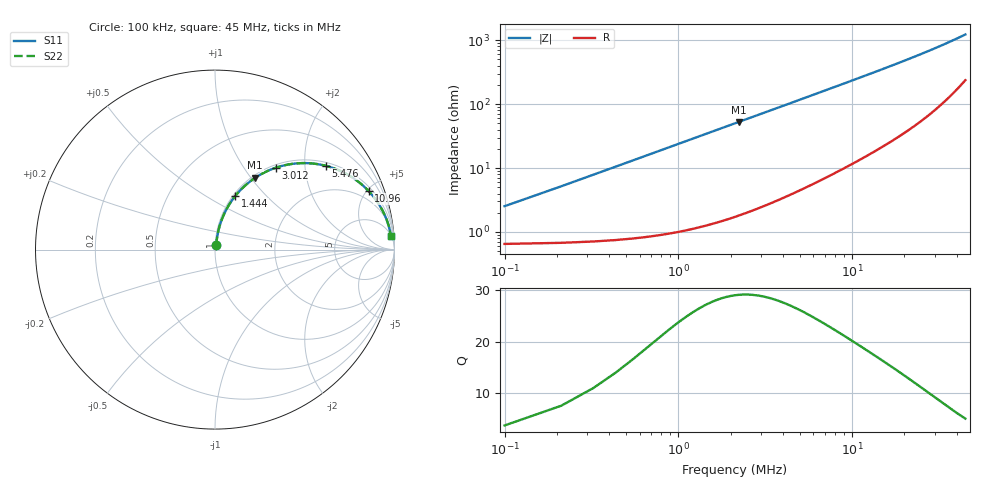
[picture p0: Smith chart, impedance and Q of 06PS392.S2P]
! Coilcraft 0603PS-392 Power Chip Inductor
! 19 February 2003
# MHZ S MA R 50
!Freq  MagS11  AngS11  MagS21  AngS21  MagS12  AngS12  MagS22  AngS22
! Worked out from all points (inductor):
!   402 points, 100 kHz to 45 MHz, reference 50 ohm
!   read as one part in series: L = 3.83 uH near 324 kHz
!   highest Q = 29.1 at 2.228 MHz (marker M1), where L = 3.75 uH
!   S11 on the Smith chart (normalised r, x): 100 kHz: 1.01, +0.05; 1.444 MHz: 1.03, +0.68; 3.012 MHz: 1.05, +1.42; 5.476 MHz: 1.10, +2.56; 10.96 MHz: 1.26, +5.12; 45 MHz: 6, +24
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0.1  0.02518 73.7  0.9932 -1.4  0.9932 -1.4  0.02518 73.7
0.212  0.05149 79.6  0.992 -2.9  0.992 -2.9  0.05149 79.6
0.436  0.1038 80.0  0.9872 -5.9  0.9872 -5.9  0.1038 80.0
0.548  0.1296 79.1  0.9838 -7.4  0.9838 -7.4  0.1296 79.1
0.66  0.155 78.1  0.9797 -8.9  0.9797 -8.9  0.155 78.1
0.772  0.1801 76.9  0.975 -10.4  0.975 -10.4  0.1801 76.9
0.996  0.2289 74.4  0.9639 -13.2  0.9639 -13.2  0.2289 74.4
1.444  0.3206 69.2  0.9355 -18.7  0.9355 -18.7  0.3206 69.2
1.78  0.3834 65.5  0.9102 -22.5  0.9102 -22.5  0.3834 65.5
2.228  0.459 60.7  0.8728 -27.3  0.8728 -27.3  0.459 60.7
3.012  0.5689 53.4  0.803 -34.6  0.803 -34.6  0.5689 53.4
4.02  0.6739 45.6  0.7149 -42.3  0.7149 -42.3  0.6739 45.6
5.476  0.7736 37.1  0.604 -50.6  0.604 -50.6  0.7736 37.1
6.484  0.8191 32.7  0.5407 -54.9  0.5407 -54.9  0.8191 32.7
7.604  0.8554 28.8  0.4817 -58.7  0.4817 -58.7  0.8554 28.8
9.172  0.8901 24.5  0.4155 -62.8  0.4155 -62.8  0.8901 24.5
10.964  0.9158 20.9  0.3572 -66.1  0.3572 -66.1  0.9158 20.9
15.108  0.9476 15.4  0.2665 -71.1  0.2665 -71.1  0.9476 15.4
22.612  0.9696 10.2  0.1781 -75.1  0.1781 -75.1  0.9696 10.2
30.116  0.9775 7.4  0.1303 -76.3  0.1303 -76.3  0.9775 7.4
37.62  0.9806 5.7  0.1002 -76.0  0.1002 -76.0  0.9806 5.7
45  0.9816 4.5  0.07979 -74.4  0.07979 -74.4  0.9816 4.5
